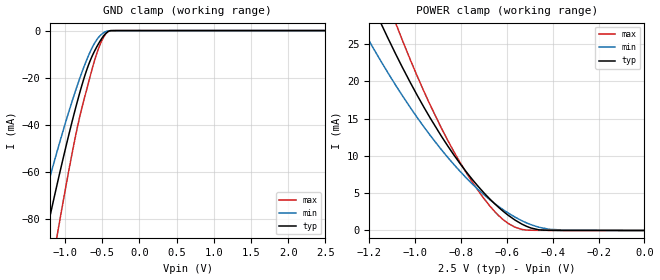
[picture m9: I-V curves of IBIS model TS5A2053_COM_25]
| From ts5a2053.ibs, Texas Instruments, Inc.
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[Model]   TS5A2053_COM_25
Model_type  Terminator
| variable   typ   min   max
C_comp   12.03pF   10.80pF   13.64pF
| C_tri-state   12.03pF   10.80pF   13.64pF
[Temperature Range]   40   100   -40
| Ambient temperature   25   85   -40
[Voltage range]   2.5   2.3   2.7
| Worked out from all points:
|   GND clamp passes 1 mA (typ) near -0.45 V on its own axis
|   POWER clamp passes 1 mA (typ) near -0.54 V on its own axis
[GND Clamp]
| TS5A2053_COM_25
|   Voltage   I(typ)   I(min)   I(max)
-5.5V     -821.7mA   -663.9mA   -1.071A
-1.395V   -106.8mA   -84.65mA   -141.4mA
-1.245V   -84.65mA   -66.83mA   -112.5mA
-1.105V   -64.81mA   -50.91mA   -86.48mA
-1.065V   -59.33mA   -46.52mA   -79.27mA
-865mV    -33.53mA   -25.98mA   -45.48mA
-755mV    -21.13mA   -16.05mA   -30.36mA
-670mV    -13.3mA    -9.456mA   -20.17mA
-565mV    -6.351mA   -3.466mA   -8.846mA
-490mV    -2.565mA   -1.09mA    -3.24mA
-420mV    -370.8uA   -115.9uA   -391.2uA
2.5V      537.1pA    627.5nA    4.067nA
[POWER Clamp]
| TS5A2053_COM_25
|   Voltage   I(typ)   I(min)   I(max)
-5.5V     630.2mA    504.2mA    817.8mA
-1.25V    34.74mA    28.13mA    42.17mA
-1.215V   32.25mA    26.19mA    38.93mA
-1.15V    27.82mA    22.73mA    33.19mA
-1.085V   23.66mA    19.47mA    27.8mA
-1.055V   21.83mA    18.04mA    25.45mA
-960mV    16.43mA    13.81mA    18.53mA
-830mV    10.08mA    8.809mA    10.51mA
-725mV    5.905mA    5.488mA    5.334mA
-615mV    2.547mA    2.762mA    1.418mA
-460mV    83.64uA    429.7uA    18.02uA
-95.1fV   537.1pA    4.231nA    12.76nA
